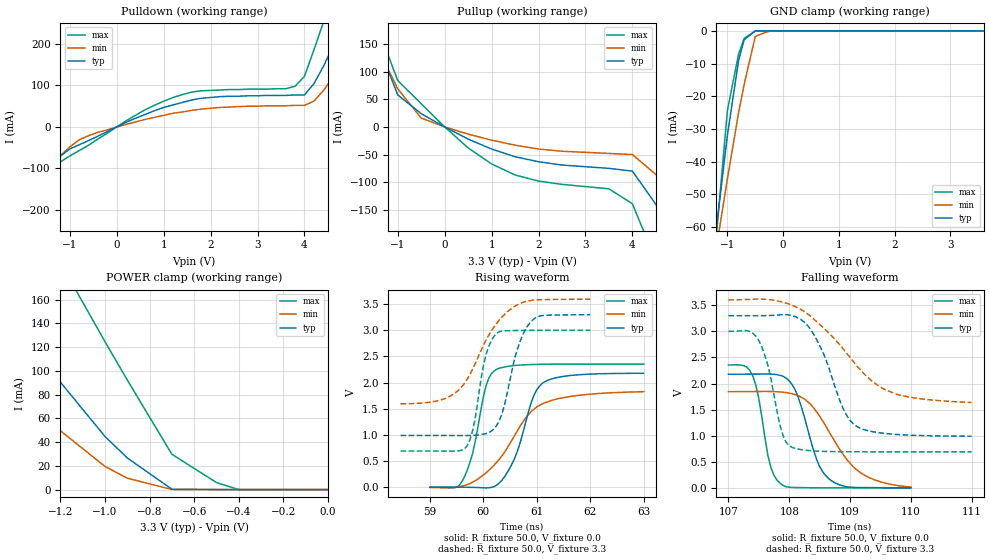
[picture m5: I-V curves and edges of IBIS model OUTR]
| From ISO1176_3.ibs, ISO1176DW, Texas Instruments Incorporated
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[Model]   OUTR
Model_type   3-state
| Signals   R
Vmeas = 2.2V   |Reference voltage for timing measurements
Cref = 15pF   |Timing specification test load capacitance value
Vref = 0   |Timing specification test load voltage; GND
| variable   typ   min   max
C_comp   2.1pF   1.7pF   2.5pF
|   typ   min   max
[Temperature Range]   25.0   -40   125
[Voltage range]   3.3V   3.6V   3.0V
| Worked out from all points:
|   slope of the pulldown table from 0 to 0.495 V, typ, clamps not added: 19.6 ohm
|   slope of the pullup table from 0 to 0.495 V, typ, clamps not added: 22.7 ohm
|   GND clamp passes 1 mA (typ) near -0.57 V on its own axis
|   POWER clamp passes 1 mA (typ) near -0.71 V on its own axis
|   rising waveform, R_fixture 50.0, V_fixture 0.0: 20-80 % time 410ps typ, 767ps min, 290ps max; typ from 0 V to 2.18 V
|   falling waveform, R_fixture 50.0, V_fixture 0.0: 20-80 % time 345ps typ, 638ps min, 215ps max; typ from 2.18 V to 0.001 V
|   rising waveform, R_fixture 50.0, V_fixture 3.3: 20-80 % time 344ps typ, 645ps min, 237ps max; typ from 0.989 V to 3.3 V
|   falling waveform, R_fixture 50.0, V_fixture 3.3: 20-80 % time 465ps typ, 950ps min, 260ps max; typ from 3.3 V to 0.991 V
[Pulldown]
|   Voltage   I(typ)  I(min)  I(max)
-3.6V     -427mA     -334mA     -572mA
-2.8V     -304mA     -244mA     -401mA
-2.4V     -243mA     -200mA     -316mA
-2V       -182mA     -155mA     -231mA
-1.2V     -70mA      -69mA      -84mA
-400mV    -22mA      -13mA      -29mA
1.4V      59mA       36mA       78mA
3.8V      77mA       52mA       98mA
4.4V      145mA      87mA       251mA
4.8V      241mA      154mA      387mA
5.4V      390mA      263mA      593mA
7.2V      850mA      600mA      1.226A
[Pullup]
|   Voltage   I(typ)  I(min)  I(max)
| Note that the[Pullup]voltage table is referenced to Vcc
| and is calculated using Vtable=Vcc - Vmeasured.
-3.6V     689mA      544mA      913mA
-2V       288mA      247mA      363mA
-1.5V     166mA      156mA      196mA
-1V       58mA       69mA       84mA
-500mV    24mA       16mA       42mA
1.5V      -54mA      -33mA      -87mA
3.5V      -75mA      -48mA      -112mA
4V        -80mA      -50mA      -139mA
4.5V      -140mA     -86mA      -242mA
5V        -217mA     -140mA     -350mA
5.5V      -295mA     -196mA     -458mA
7.2V      -562mA     -390mA     -830mA
[GND_clamp]
|   Voltage   I(typ)   I(min)   I(max)
| Outputs in High Impedance (off)
-3.6V     -425.9mA   -334mA     -570.9mA
-1.2V     -60.51mA   -66.54mA   -62.98mA
-1.1V     -46.2mA    -55.88mA   -43.66mA
-1V       -31.9mA    -45.23mA   -24.35mA
-800mV    -9.097mA   -25.09mA   -7.168mA
-700mV    -2.72mA    -16.39mA   -2.309mA
-500mV    -16.68uA   -1.726mA   -51.55uA
-300mV    -3.339uA   -347.5uA   -10.31uA
-200mV    -4.168nA   -2.232uA   -2.942nA
3.6V      8.784nA    32.33nA    5.263uA
[POWER_clamp]
|   Voltage  I(typ)   I(min)   I(max)
| Note that the [POWER_clamp] voltage table is referenced to Vcc
| and is calculated using Vtable = Vcc - Vmeasured.
| Outputs in Tri-state.
-3.6V     688.9mA    487.5mA    1.016A
-1.9V     261.9mA    173.3mA    429.5mA
-1.8V     237.1mA    155.1mA    395.2mA
-1.5V     163.1mA    101.4mA    292.7mA
-1.2V     90.4mA     49.49mA    191mA
-1.1V     67.54mA    34.49mA    157.7mA
-1V       44.68mA    19.49mA    124.5mA
-900mV    26.67mA    9.609mA    92.23mA
-700mV    313.1uA    71.19uA    29.75mA
-500mV    62.63uA    14.3uA     5.96mA
-400mV    17.51nA    62.62nA    10.53uA
0V        50.28pA    1.949nA    141.4pA
[Ramp]
|   typ   min   max
dV/dt_r   1.88V/.33ns   1.48V/.58ns   1.81V/.23ns
dV/dt_f   1.92V/.36ns   1.67V/.60ns   2.07V/.23ns
R_load = 50
[Rising Waveform]
R_fixture = 50.0
V_fixture = 0.0
C_fixture = 0p
L_fixture = 0n
|   V(typ)   V(min)   V(max)
59ns      -7.749uV   -5.606mV   288.9uV
59.6ns    -109.3uV   19.92mV    107.1mV
59.8ns    -3.444mV   95mV       650.6mV
60.05ns   -12.83mV   275mV      1.934V
60.25ns   39.93mV    475.7mV    2.256V
60.55ns   472.4mV    926.2mV    2.323V
60.9ns    1.631V     1.452V     2.345V
61.1ns    1.985V     1.59V      2.35V
61.65ns   2.138V     1.738V     2.354V
63ns      2.178V     1.826V     2.354V
[Falling Waveform]
R_fixture = 50.0
V_fixture = 0.0
C_fixture = 0p
L_fixture = 0n
|   V(typ)   V(min)   V(max)
107ns     2.179V     1.844V     2.355V
107.4ns   2.18V      1.846V     2.146V
107.5ns   2.181V     1.847V     1.708V
107.7ns   2.181V     1.847V     384.7mV
107.9ns   2.138V     1.833V     46.95mV
108.1ns   1.873V     1.786V     6.564mV
108.4ns   547.8mV    1.458V     1.337mV
108.6ns   175.4mV    1.088V     499.6uV
109.2ns   5.764mV    269.8mV    10.24uV
110ns     850.1uV    16.75mV    -11.17uV
[Rising Waveform]
R_fixture = 50.0
V_fixture = 3.3
V_fixture_min = 3.6
V_fixture_max = 3.0
C_fixture = 0p
L_fixture = 0n
|   V(typ)   V(min)  V(max)
58.45ns   989mV      1.596V     691mV
59.3ns    989mV      1.701V     690mV
59.7ns    987mV      2.069V     798mV
59.8ns    990mV      2.26V      1.083V
60.05ns   1.025V     2.813V     2.536V
60.25ns   1.182V     3.133V     2.943V
60.4ns    1.592V     3.307V     2.992V
60.65ns   2.681V     3.494V     2.996V
60.85ns   3.115V     3.562V     2.998V
62ns      3.298V     3.596V     3V
[Falling Waveform]
R_fixture = 50.0
V_fixture = 3.3
V_fixture_min = 3.6
V_fixture_max = 3.0
C_fixture = 0p
L_fixture = 0n
|   V(typ)   V(min)  V(max)
107ns     3.3V       3.602V     3V
107.5ns   3.3V       3.618V     2.824V
107.7ns   3.303V     3.612V     2.344V
107.9ns   3.321V     3.558V     995mV
108.1ns   3.301V     3.499V     774mV
108.4ns   2.949V     3.24V      708mV
108.9ns   1.491V     2.647V     693mV
109.1ns   1.185V     2.355V     692mV
109.8ns   1.021V     1.783V     691mV
111ns     991mV      1.637V     691mV
